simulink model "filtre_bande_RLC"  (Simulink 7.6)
settings: Solver=ode45  StartTime=0.0  StopTime=10.0  RelTol=1e-3
libraries: fl_lib x10

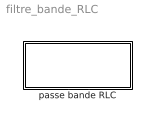
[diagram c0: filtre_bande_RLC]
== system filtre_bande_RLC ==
  passe bande RLC : Subsystem

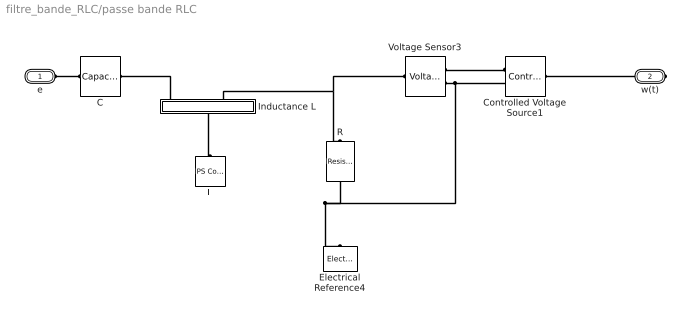
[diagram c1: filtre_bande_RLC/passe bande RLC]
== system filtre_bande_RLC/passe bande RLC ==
  C : fl_lib/Electrical/Electrical Elements/Capacitor  DialogController=NetworkEngine.DynNeDlgSource  SystemSampleTime=-1  c=1e-6 F  v0=0 V  r=1e-6 Ohm  g=0 1/Ohm  i_Log=off  v_Log=off  vc_Log=off  LocalVarNames=|i|v|vc  LocalVarDescs=|i|v|Internal variable for voltage across capacitor term  LocalVarLogging=[0 0 0]
  Controlled Voltage Source1 : fl_lib/Electrical/Electrical Sources/Controlled Voltage Source  DialogController=NetworkEngine.DynNeDlgSource  SystemSampleTime=-1  i_Log=off  v_Log=off  LocalVarNames=|i|v  LocalVarDescs=|i|v  LocalVarLogging=[0 0]
  Electrical Reference4 : fl_lib/Electrical/Electrical Elements/Electrical Reference  DialogController=NetworkEngine.DynNeDlgSource  SystemSampleTime=-1  i_Log=off  LocalVarNames=|i  LocalVarDescs=|i  LocalVarLogging=0
  "Inductance L  " : Subsystem  mask{L=0}
      mask prompts: L "Inductance"
  L : fl_lib/Physical Signals/Sources/PS Constant  DialogController=NetworkEngine.DynNeDlgSource  SystemSampleTime=-1  constant=L  LocalVarLogging=[]
  R : fl_lib/Electrical/Electrical Elements/Resistor  DialogController=NetworkEngine.DynNeDlgSource  SystemSampleTime=-1  R=1 Ohm  i_Log=off  v_Log=off  LocalVarNames=|i|v  LocalVarDescs=|i|v  LocalVarLogging=[0 0]
  Voltage Sensor3 : fl_lib/Electrical/Electrical Sensors/Voltage Sensor  DialogController=NetworkEngine.DynNeDlgSource  SystemSampleTime=-1  i1_Log=off  v1_Log=off  LocalVarNames=|i1|v1  LocalVarDescs=|i1|v1  LocalVarLogging=[0 0]
  e : PMIOPort  Port=1  Side=Left
  w(t) : PMIOPort  Port=2  Side=Right
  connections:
  C/RConn1 -- "Inductance L  "/RConn1
  Voltage Sensor3/RConn2 -- R/RConn1 -- Electrical Reference4/LConn1 -- Controlled Voltage Source1/RConn2
  "Inductance L  "/LConn1 -- L/RConn1
  "Inductance L  "/RConn2 -- R/LConn1 -- Voltage Sensor3/LConn1
  e/RConn1 -- C/LConn1
  Voltage Sensor3/RConn1 -- Controlled Voltage Source1/RConn1
  Controlled Voltage Source1/LConn1 -- w(t)/RConn1

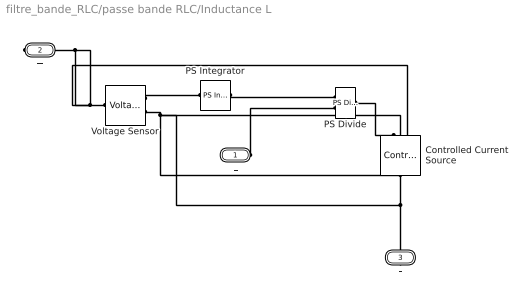
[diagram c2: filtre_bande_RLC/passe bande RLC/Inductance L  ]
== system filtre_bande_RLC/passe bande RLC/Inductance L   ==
  Controlled Current Source : fl_lib/Electrical/Electrical Sources/Controlled Current Source  DialogController=NetworkEngine.DynNeDlgSource  SystemSampleTime=-1  i_Log=off  v_Log=off  LocalVarNames=|i|v  LocalVarDescs=|i|v  LocalVarLogging=[0 0]
  PS Divide : fl_lib/Physical Signals/Functions/PS Divide  DialogController=NetworkEngine.DynNeDlgSource  SystemSampleTime=-1  LocalVarLogging=[]
  PS Integrator : fl_lib/Physical Signals/Linear Operators/PS Integrator  DialogController=NetworkEngine.DynNeDlgSource  SystemSampleTime=-1  x0=0  x_Log=off  LocalVarNames=|x  LocalVarDescs=|x  LocalVarLogging=0
  Voltage Sensor : fl_lib/Electrical/Electrical Sensors/Voltage Sensor  DialogController=NetworkEngine.DynNeDlgSource  SystemSampleTime=-1  i1_Log=off  v1_Log=off  LocalVarNames=|i1|v1  LocalVarDescs=|i1|v1  LocalVarLogging=[0 0]
  L : PMIOPort  Port=1  Side=Left
  + : PMIOPort  Port=2  Side=Right
  - : PMIOPort  Port=3  Side=Right
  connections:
  Voltage Sensor/RConn2 -- Controlled Current Source/LConn1 -- -/RConn1
  L/RConn1 -- PS Divide/LConn2
  Voltage Sensor/RConn1 -- PS Integrator/LConn1
  PS Integrator/RConn1 -- PS Divide/LConn1
  Voltage Sensor/LConn1 -- +/RConn1 -- Controlled Current Source/RConn2
  PS Divide/RConn1 -- Controlled Current Source/RConn1
